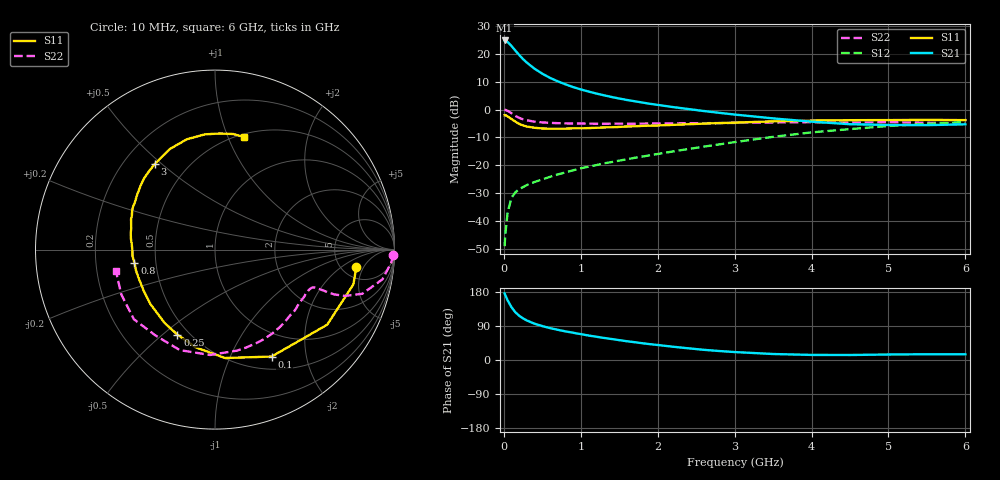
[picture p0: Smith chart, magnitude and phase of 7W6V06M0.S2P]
! Infineon Technologies  Discrete & RF Semiconductors
! BFS17W
! Si NPN RF Bipolar Junction Transistor in SOT323
! VCE = 6 V  IC = 6 mA
! Common Emitter S-Parameters:  August  1999
# GHz  S  MA  R  50
!  f  S11  S21  S12  S22
! GHz  MAG  ANG  MAG  ANG  MAG  ANG  MAG  ANG
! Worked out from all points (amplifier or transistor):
!   36 points, 10 MHz to 6 GHz, reference 50 ohm
!   highest |S21| = 24.7 dB at 10 MHz (marker M1)
!   |S21| within 3 dB of that: start of sweep to 130.7 MHz
!   unconditionally stable (mu >= 1): 528.3 MHz to 2.395 GHz; 5.108 GHz to end of sweep
!   at 250 MHz: K = 0.64, MSG = 22.9 dB, |S12| = -27.7 dB
!   at 1.4 GHz: K = 1.21, MAG = 8.9 dB, |S12| = -18.8 dB
!   at 6 GHz: K = 1.06, MAG = -1.9 dB, |S12| = -4.5 dB
!   S11 on the Smith chart (normalised r, x): 10 MHz: 6.84, -3.52; 100 MHz: 0.66, -1.45; 250 MHz: 0.43, -0.56; 800 MHz: 0.38, -0.07; 3 GHz: 0.33, +0.47; 6 GHz: 0.53, +1.14
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0.01  0.7935 -6.9  17.18 175.6  0.0036 84.6  0.9943 -1.7
0.02  0.795 -14.1  17.07 170.5  0.006 83.3  0.9844 -4.3
0.05  0.7522 -33.8  16.08 157.1  0.0147 74.8  0.9472 -10.1
0.1  0.6742 -62.1  13.66 139.3  0.0265 63.2  0.8565 -16.7
0.15  0.6067 -84.7  11.31 125.9  0.033 55.6  0.7692 -19.6
0.2  0.5554 -101.1  9.436 116.7  0.0379 53.6  0.7098 -20.6
0.25  0.5178 -113.9  7.968 109.7  0.041 51.3  0.6674 -20.7
0.3  0.4963 -124.3  6.877 104.2  0.0447 51.1  0.6411 -20.7
0.4  0.4711 -139.6  5.359 95.7  0.0506 52.4  0.6056 -20.7
0.5  0.4583 -150.4  4.374 89.5  0.0564 54.4  0.5889 -20.9
0.6  0.4541 -158.5  3.682 84.2  0.0626 56.6  0.5775 -21.7
0.8  0.4548 -170.6  2.824 75.6  0.075 59.6  0.5656 -24.4
0.9  0.4611 -175.5  2.524 71.9  0.0818 61.1  0.5617 -26.0
1.1  0.4653 176.0  2.097 64.6  0.0949 63.3  0.5592 -29.7
1.3  0.4783 169.0  1.798 58.3  0.1091 64.7  0.5564 -34.0
1.6  0.4979 160.0  1.481 49.5  0.129 66.7  0.5567 -40.6
2.2  0.5314 144.5  1.106 35.0  0.178 69.6  0.5661 -55.8
3  0.583 125.2  0.813 21.0  0.2613 68.6  0.576 -77.7
3.5  0.6142 114.2  0.694 15.8  0.325 65.3  0.5878 -92.7
4.5  0.6447 95.0  0.546 13.2  0.4463 53.5  0.582 -124.8
5.5  0.652 80.9  0.526 15.2  0.5536 40.4  0.5788 -154.4
6  0.6469 75.5  0.544 15.1  0.596 33.9  0.5647 -167.6
